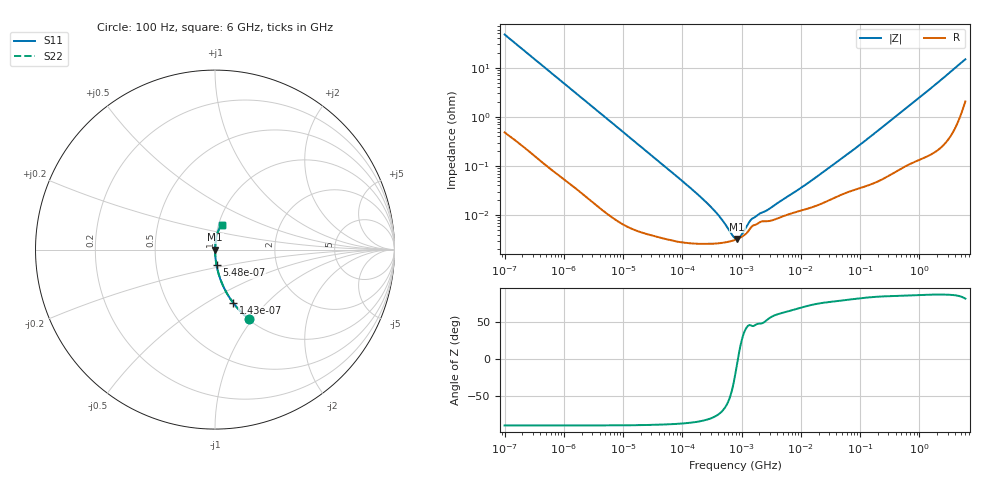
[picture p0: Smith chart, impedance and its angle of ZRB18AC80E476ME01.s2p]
!Murata Part Number: ZRB18AC80E476ME01
!These Parameters are Measured in Series Mode Connection
!Data Generated on Jun 10, 2025
!  o--ll--o
!Port1  Port2
!  o------o
!Operation Temp=25[degC], DC Bias Voltage=0[V]
!Freq. Start=100[Hz] Stop=6[GHz] 401[Steps]
# Hz S RI R 50
!Freq.(Hz) S11(Real) S11(Imag) S21(Real) S21(Imag) S12(Real) S12(Imag) S22(Real) S22(Imag)
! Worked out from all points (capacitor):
!   401 points, 100 Hz to 6 GHz, reference 50 ohm
!   read as one part in series: C = 33.3 uF near 109 Hz
!   lowest |Z| = 3.25 mohm at 847.2 kHz (marker M1)
!   series resonance near 866.2 kHz, so ESL is about 1 nH
!   S11 on the Smith chart (normalised r, x): 100 Hz: 1.01, -0.95; 143 Hz: 1.01, -0.67; 548 Hz: 1.00, -0.18; 6 GHz: 1.04, +0.29
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100  0.1876 -0.3854  0.8124 0.3854  0.8124 0.3854  0.1876 -0.3854
143  0.1029 -0.2986  0.8971 0.2986  0.8971 0.2986  0.1029 -0.2986
187  0.0637 -0.2389  0.9363 0.2389  0.9363 0.2389  0.0637 -0.2389
280  0.0302 -0.166  0.9698 0.166  0.9698 0.166  0.0302 -0.166
548  0.0086 -0.0872  0.9914 0.0872  0.9914 0.0872  0.0086 -0.0872
981  0.00297 -0.0492  0.997 0.0492  0.997 0.0492  0.00297 -0.0492
2008  0.000862 -0.0242  0.9991 0.0242  0.9991 0.0242  0.000862 -0.0242
40335  3.66e-05 -0.00122  1 0.00122  1 0.00122  3.66e-05 -0.00122
169018  2.61e-05 -0.000284  1 0.000284  1 0.000284  2.61e-05 -0.000284
252896  2.58e-05 -0.00018  1 0.00018  1 0.00018  2.58e-05 -0.00018
395726  2.64e-05 -9.96e-05  1 9.96e-05  1 9.96e-05  2.64e-05 -9.96e-05
452617  2.69e-05 -8e-05  1 8e-05  1 8e-05  2.69e-05 -8e-05
774597  3.11e-05 -1.28e-05  1 1.28e-05  1 1.28e-05  3.11e-05 -1.28e-05
847162  3.24e-05 -2.5e-06  1 2.5e-06  1 2.5e-06  3.24e-05 -2.5e-06
1734173  6.36e-05 6.79e-05  0.9999 -6.79e-05  0.9999 -6.79e-05  6.36e-05 6.79e-05
2481164  7.47e-05 9.22e-05  0.9999 -9.22e-05  0.9999 -9.22e-05  7.47e-05 9.22e-05
1.555665e7  0.000144 0.000495  0.9999 -0.000495  0.9999 -0.000495  0.000144 0.000495
8.154455e7  0.000332 0.00222  0.9997 -0.00222  0.9997 -0.00222  0.000332 0.00222
3.124326e8  0.000704 0.00799  0.9993 -0.00799  0.9993 -0.00799  0.000704 0.00799
1.791126e9  0.00375 0.0433  0.9962 -0.0433  0.9962 -0.0433  0.00375 0.0433
5.016141e9  0.0256 0.1198  0.9744 -0.1198  0.9744 -0.1198  0.0256 0.1198
6e9  0.0402 0.1383  0.9598 -0.1383  0.9598 -0.1383  0.0402 0.1383
